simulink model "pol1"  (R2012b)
settings: Solver=ode45  StartTime=0.0  StopTime=10.0  RelTol=1e-3
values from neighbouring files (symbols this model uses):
  k1 = 100    [aktiv_tilger_1.m]    (also in aktiv_tilger_12.m; aktiv_tilger_2.m = 5; aktiv_tilger_3.m; aktiv_tilger_31.m)
  k2 = 10    [aktiv_tilger_1.m]    (also in aktiv_tilger_12.m; aktiv_tilger_2.m = 10,      c2 = 10; aktiv_tilger_3.m; aktiv_tilger_31.m)
  T1 = 1    [PID_windup1.m]    (also in pol_1.m = -5; pol_2.m = -5; pol_3.m = -5; sprung.m = x(2))
  T2 = 5    [PID_windup1.m]    (also in pol_1.m = 10; pol_2.m = 10; pol_3.m = 10; sprung.m = x(3))

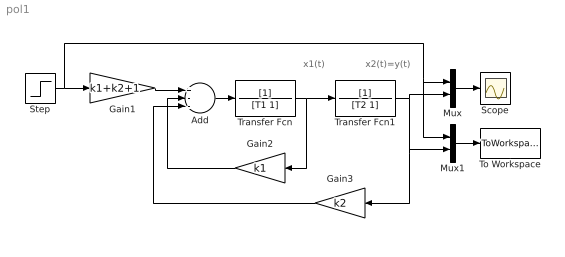
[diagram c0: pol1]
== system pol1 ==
  note: x2(t)=y(t)
  note: x1(t)
  Add : Sum  Inputs=+--
  Gain1 : Gain  Gain=k1+k2+1
  Gain2 : Gain  Gain=k1
  Gain3 : Gain  Gain=k2
  Mux : Mux  Inputs=2
  Mux1 : Mux  Inputs=2
  Scope : Scope
  Step : Step  SampleTime=0
  To Workspace : ToWorkspace  VariableName=y  SampleTime=-1  SaveFormat=Structure With Time
  Transfer Fcn : TransferFcn  Denominator=[T1 1]
  Transfer Fcn1 : TransferFcn  Denominator=[T2 1]
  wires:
  Add/1 -> Transfer Fcn/1
  Gain1/1 -> Add/1
  Transfer Fcn/1 -> Gain2/1, Transfer Fcn1/1
  Gain2/1 -> Add/2
  Gain3/1 -> Add/3
  Transfer Fcn1/1 -> Mux/2, Mux1/2, Gain3/1
  Mux/1 -> Scope/1
  Step/1 -> Mux1/1, Mux/1, Gain1/1
  Mux1/1 -> To Workspace/1
